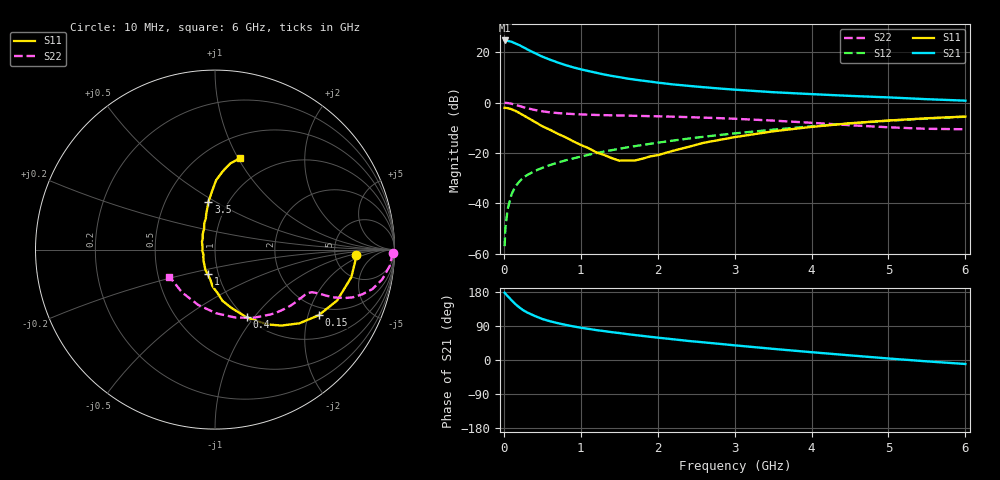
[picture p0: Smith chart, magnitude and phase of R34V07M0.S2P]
! SIEMENS Small Signal Semiconductors
! BFR181
! Si NPN RF Bipolar Junction Transistor in SOT23
! VCE = 4 V  IC = 7 mA
! Common Emitter S-Parameters:  May  1996
# GHz  S  MA  R  50
!  f  S11  S21  S12  S22
! GHz  MAG  ANG  MAG  ANG  MAG  ANG  MAG  ANG
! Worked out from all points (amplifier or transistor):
!   36 points, 10 MHz to 6 GHz, reference 50 ohm
!   highest |S21| = 24.7 dB at 10 MHz (marker M1)
!   |S21| within 3 dB of that: start of sweep to 272.5 MHz
!   unconditionally stable (mu >= 1): 943.6 MHz to 2.827 GHz
!   at 250 MHz: K = 0.51, MSG = 26.0 dB, |S12| = -29.9 dB
!   at 1.4 GHz: K = 1.05, MAG = 13.4 dB, |S12| = -18.9 dB
!   at 6 GHz: K = 0.86, MSG = 3.2 dB, |S12| = -5.6 dB
!   S11 on the Smith chart (normalised r, x): 10 MHz: 8.12, -1.34; 150 MHz: 1.70, -2.34; 400 MHz: 1.01, -0.92; 1 GHz: 0.89, -0.25; 3.5 GHz: 0.81, +0.46; 6 GHz: 0.72, +1.02
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0.01  0.786 -2.3  17.15 177.4  0.0014 84.1  0.9891 -1.0
0.02  0.7841 -4.7  16.89 175.0  0.0032 89.7  0.9868 -2.2
0.05  0.7751 -11.4  16.8 168.5  0.0077 82.6  0.9779 -5.3
0.1  0.7372 -22.6  16.18 157.8  0.015 79.5  0.9464 -10.1
0.15  0.6833 -32.4  14.96 147.5  0.0215 73.7  0.9038 -14.1
0.2  0.6245 -41.1  13.88 139.1  0.0267 71.8  0.8575 -16.9
0.25  0.5624 -48.8  12.67 131.6  0.032 68.5  0.8125 -19.1
0.3  0.5093 -55.0  11.52 125.8  0.036 67.5  0.774 -20.4
0.4  0.4162 -65.0  9.665 116.4  0.0436 66.0  0.7148 -21.9
0.5  0.3379 -74.2  8.183 108.2  0.0503 65.9  0.6707 -22.5
0.6  0.2884 -81.7  7.121 102.3  0.0573 66.0  0.6392 -22.8
0.7  0.2404 -86.9  6.269 97.3  0.064 66.4  0.6187 -23.1
0.8  0.205 -94.0  5.565 92.8  0.0708 66.6  0.603 -23.4
1  0.1437 -106.2  4.589 85.2  0.0843 67.3  0.5821 -24.2
1.1  0.1246 -115.6  4.232 82.2  0.0917 67.4  0.5743 -24.9
1.3  0.0914 -133.8  3.624 76.3  0.1061 67.4  0.5627 -26.3
1.6  0.0707 -174.8  3.012 68.3  0.1285 66.6  0.5503 -29.2
2.2  0.1101 128.4  2.295 54.7  0.1756 64.1  0.5241 -36.6
3.5  0.2682 97.8  1.608 29.4  0.2892 54.4  0.4384 -59.8
4.5  0.3878 89.0  1.357 12.2  0.3865 43.8  0.355 -88.8
5.5  0.4877 79.9  1.167 -3.6  0.4808 31.2  0.3011 -127.7
6  0.5277 74.8  1.091 -10.5  0.5233 24.2  0.2949 -149.4
